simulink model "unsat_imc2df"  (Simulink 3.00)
settings: Solver=ode45  SolverMode=SingleTasking  StartTime=0.0  StopTime=50  FixedStep=st_size  MaxStep=st_size  RelTol=1e-5  AbsTol=1e-6
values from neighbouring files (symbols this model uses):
  Disturb = Setpoint    [mimo_MSF1DF_sim.m]    (also in mimo_MSF2DF_sim.m)
  Setpoint = zeros(1,n)    [mimo_MSF1DF_sim.m]    (also in mimo_MSF2DF_sim.m)
undefined symbols (not defined in the file or in its folder): denCs, denCs2, denMs, denPd, denPs, numCs, numCs2, numMs, numPd, numPs, Qdden, Qdnum
libraries: MIMO_lib x2

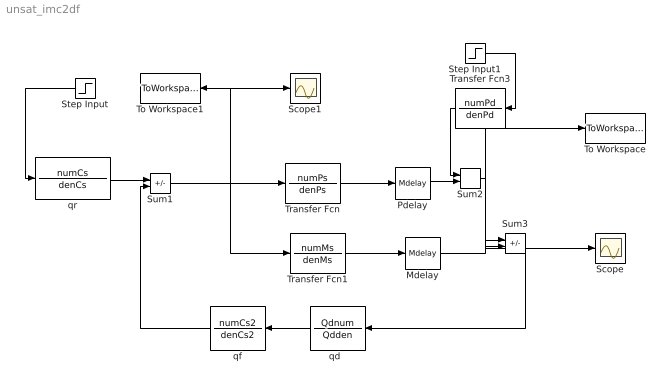
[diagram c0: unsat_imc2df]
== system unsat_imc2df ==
  Mdelay : MIMO_lib/Mdelay  Mdelay=Mdelay
  Pdelay : MIMO_lib/Mdelay  Mdelay=Pdelay
  Scope : Scope
  Scope1 : Scope
  Step Input : Step  Orientation=left  Time=0  Before=0  After=Setpoint  SampleTime=0
  Step Input1 : Step  Time=0  Before=0  After=Disturb  SampleTime=0
  Sum1 : Sum  Inputs=+-  SaturateOnIntegerOverflow=on
  Sum2 : Sum  Inputs=++  SaturateOnIntegerOverflow=on
  Sum3 : Sum  Inputs=+-  SaturateOnIntegerOverflow=on
  To Workspace : ToWorkspace  VariableName=simout  SampleTime=-1  SaveFormat=Matrix
  To Workspace1 : ToWorkspace  VariableName=effort  SampleTime=-1  SaveFormat=Matrix
  Transfer Fcn : TransferFcn  Numerator=numPs  Denominator=denPs
  Transfer Fcn1 : TransferFcn  Numerator=numMs  Denominator=denMs
  Transfer Fcn3 : TransferFcn  Orientation=left  Numerator=numPd  Denominator=denPd
  "qd  " : TransferFcn  Orientation=left  Numerator=Qdnum  Denominator=Qdden
  qf : TransferFcn  Orientation=left  Numerator=numCs2  Denominator=denCs2
  qr : TransferFcn  Numerator=numCs  Denominator=denCs
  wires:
  Step Input/1 -> qr/1
  Transfer Fcn/1 -> Pdelay/1
  Pdelay/1 -> Sum2/2
  qr/1 -> Sum1/1
  Transfer Fcn1/1 -> Mdelay/1
  Sum2/1 -> Sum3/1, Scope/1, To Workspace/1
  Mdelay/1 -> Sum3/2
  Sum3/1 -> "qd  "/1
  "qd  "/1 -> qf/1
  qf/1 -> Sum1/2
  Transfer Fcn3/1 -> Sum2/1
  Step Input1/1 -> Transfer Fcn3/1
  Sum1/1 -> Transfer Fcn/1, Transfer Fcn1/1, Scope1/1, To Workspace1/1
